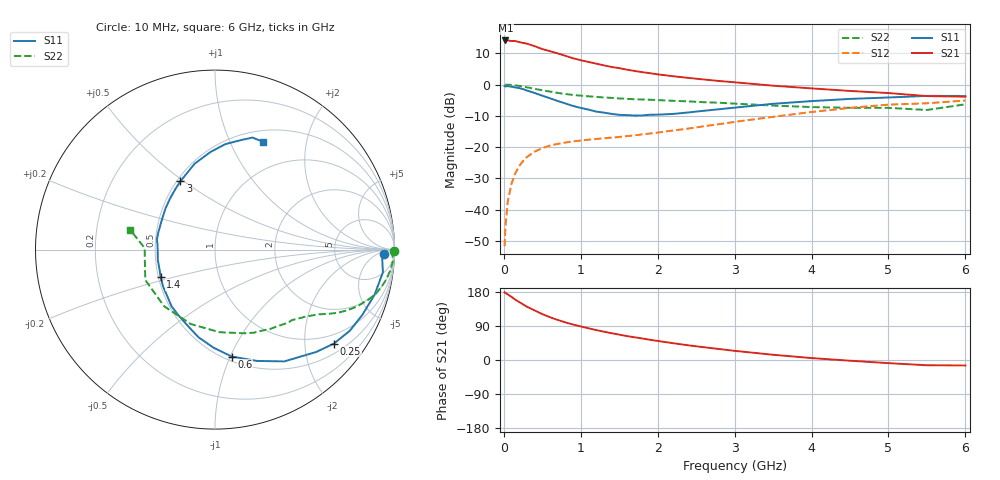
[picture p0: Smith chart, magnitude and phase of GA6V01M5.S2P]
! Infineon Technologies  Discrete & RF Semiconductors
! BF775
! Si NPN RF Bipolar Junction Transistor in SOT23
! VCE = 6 V  IC = 1.5 mA
! Common Emitter S-Parameters:  May  1996
# GHz  S  MA  R  50
!  f  S11  S21  S12  S22
! GHz  MAG  ANG  MAG  ANG  MAG  ANG  MAG  ANG
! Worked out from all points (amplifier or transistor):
!   36 points, 10 MHz to 6 GHz, reference 50 ohm
!   highest |S21| = 14.1 dB at 20 MHz (marker M1)
!   |S21| within 3 dB of that: start of sweep to 536 MHz
!   unconditionally stable (mu >= 1): 1.319 GHz to 3.495 GHz
!   at 250 MHz: K = 0.24, MSG = 18.9 dB, |S12| = -24.5 dB
!   at 1.4 GHz: K = 1.04, MAG = 10.1 dB, |S12| = -17.0 dB
!   at 6 GHz: K = 0.97, MSG = 0.6 dB, |S12| = -5.1 dB
!   S11 on the Smith chart (normalised r, x): 10 MHz: 28, -13; 250 MHz: 0.74, -2.70; 600 MHz: 0.54, -1.01; 1.4 GHz: 0.51, -0.18; 3 GHz: 0.52, +0.49; 6 GHz: 0.64, +1.34
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0.01  0.9425 -1.6  5.019 178.9  0.0026 91.2  0.999 -0.6
0.02  0.9331 -3.2  5.072 177.0  0.0052 89.0  0.9874 -1.2
0.05  0.9441 -7.7  5.071 173.2  0.0134 87.3  0.9941 -3.4
0.1  0.9239 -15.8  4.979 166.6  0.026 80.0  0.9845 -6.6
0.15  0.898 -23.9  4.965 159.0  0.0382 75.7  0.969 -9.8
0.25  0.8446 -38.3  4.631 146.7  0.0598 67.6  0.9294 -15.3
0.3  0.8022 -45.3  4.505 140.6  0.0693 64.4  0.9034 -17.7
0.4  0.733 -58.2  4.111 130.8  0.0844 58.0  0.8543 -21.7
0.5  0.6631 -69.3  3.693 121.1  0.0963 53.1  0.81 -24.7
0.6  0.6032 -81.1  3.416 112.9  0.1059 49.5  0.7714 -27.1
0.8  0.4978 -100.5  2.878 99.3  0.1182 44.8  0.7057 -30.6
0.9  0.4546 -108.8  2.634 93.6  0.1232 43.6  0.6818 -31.9
1.1  0.3978 -127.5  2.298 83.7  0.1313 42.1  0.6486 -34.6
1.4  0.3394 -153.3  1.911 70.7  0.1414 42.3  0.6116 -38.5
1.7  0.3197 -177.1  1.65 59.9  0.1538 44.5  0.5814 -42.6
2.2  0.3387 151.3  1.358 44.3  0.184 47.4  0.5493 -51.2
3  0.4271 116.8  1.087 24.2  0.2527 47.9  0.4954 -70.3
3.5  0.492 103.3  0.959 13.8  0.3048 45.0  0.461 -86.8
4.5  0.5894 84.6  0.79 -1.9  0.424 33.6  0.4243 -132.0
5  0.621 77.8  0.731 -8.3  0.4768 25.8  0.4237 -156.5
5.5  0.6583 71.5  0.654 -13.9  0.5017 16.7  0.3922 178.7
6  0.6575 65.8  0.639 -14.4  0.5552 12.0  0.483 167.1
